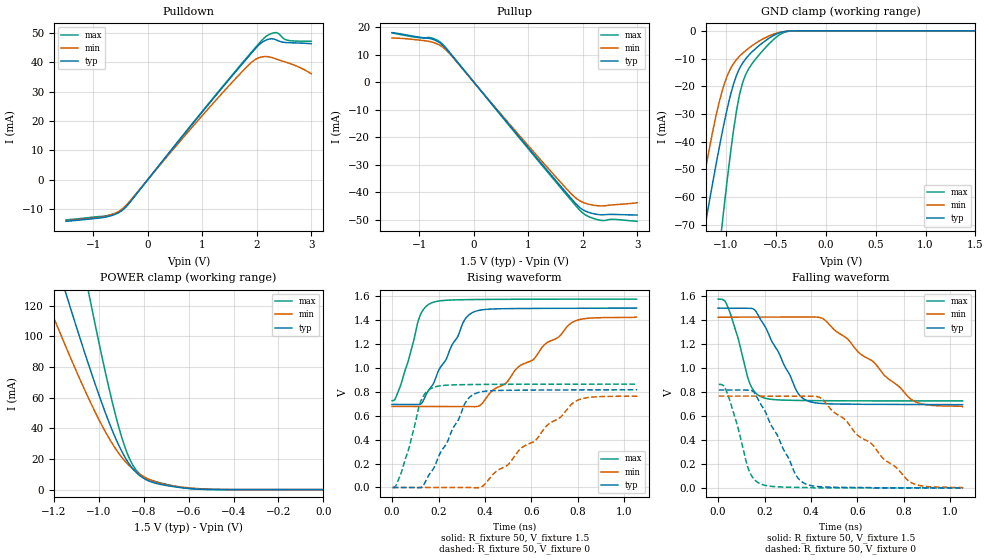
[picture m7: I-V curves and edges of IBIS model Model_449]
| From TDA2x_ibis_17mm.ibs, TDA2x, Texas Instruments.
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| Model based on original model for DDR_DIFFIOPB_H
|   Sub model SR100_DRV40_1P5
[model]   Model_449
|[Description]  [1.5V-I/O-X-X]
|   , ,
|[Input Load]
|[Output Drive]
|Voltage   1.5V
|Mode   I/O
Model_type   I/O
Polarity   Non-Inverting
Enable   Active-Low
Vinl =  0.65
Vinh =  0.85
Cref =  15.0000pF
Rref =  100.0000M
Vref =  0V
Vmeas =  0.75
C_comp   2p   2p   2p
[Model Spec]
Vinl   0.65   0.6125   0.6875
Vinh   0.85   0.8125   0.8875
[Receiver Thresholds]
Tslew_ac = 0.5n
Vth= 0.75
Vth_max= 0.7875
Vth_min= 0.675
Vinh_ac= 0.175
Vinh_dc= 0.1
Vinl_ac= -0.175
Vinl_dc= -0.1
[Temperature Range]   25   125   -40
[Voltage Range]   1.5   1.425   1.575
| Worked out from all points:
|   slope of the pulldown table from 0 to 0.225 V, typ, clamps not added: 43 ohm
|   slope of the pullup table from 0 to 0.225 V, typ, clamps not added: 41.7 ohm
|   GND clamp passes 1 mA (typ) near -0.48 V on its own axis
|   POWER clamp passes 1 mA (typ) near -0.62 V on its own axis
|   rising waveform, R_fixture 50, V_fixture 1.5: 20-80 % time 123ps typ, 282ps min, 71.2ps max; typ from 0.695 V to 1.5 V
|   rising waveform, R_fixture 50, V_fixture 0: 20-80 % time 123ps typ, 273ps min, 71.1ps max; typ from 0 V to 0.817 V
|   falling waveform, R_fixture 50, V_fixture 1.5: 20-80 % time 122ps typ, 255ps min, 70.8ps max; typ from 1.5 V to 0.695 V
|   falling waveform, R_fixture 50, V_fixture 0: 20-80 % time 123ps typ, 263ps min, 71.1ps max; typ from 0.817 V to 0 V
[POWER_clamp]
-1.5V     302.8mA    223.9mA    484.4mA
-1.242V   174.3mA    127.3mA    279.1mA
-1.136V   123.3mA    89.68mA    196.8mA
-1.045V   81.65mA    59.62mA    128.8mA
-1.03V    75mA       54.92mA    117.8mA
-939.4mV  38.44mA    29.91mA    56.84mA
-893.9mV  23.93mA    20.41mA    32.31mA
-848.5mV  13.61mA    13.43mA    15.91mA
-803mV    7.623mA    8.663mA    8.564mA
-712.1mV  3.022mA    3.561mA    3.877mA
-575.8mV  470.5uA    872uA      449uA
0V        112.6nA    435.6nA    613.8nA
[Pulldown]
-1.5V     -14.18mA   -14.05mA   -13.7mA
-727.3mV  -12.54mA   -12.27mA   -12.15mA
-545.5mV  -11.35mA   -10.95mA   -11.1mA
-409.1mV  -9.378mA   -8.925mA   -9.416mA
1.227V    28.16mA    26.58mA    28.43mA
1.818V    41.23mA    38.42mA    41.56mA
2V        45.11mA    41.2mA     45.49mA
2.182V    47.62mA    41.92mA    48.94mA
2.273V    47.99mA    41.65mA    49.78mA
2.364V    47.57mA    41.06mA    50.1mA
2.545V    46.7mA     39.96mA    47.58mA
3V        46.28mA    36.09mA    47.12mA
[Pullup]
-1.5V     17.97mA    16.01mA    17.82mA
-1V       16.28mA    15.23mA    16.1mA
-772.7mV  15.66mA    14.54mA    16.02mA
-590.9mV  13.75mA    12.97mA    14.08mA
-409.1mV  9.799mA    9.534mA    9.955mA
1.409V    -33.42mA   -32.26mA   -33.94mA
1.773V    -41.87mA   -40.19mA   -42.52mA
1.909V    -44.87mA   -42.6mA    -45.68mA
2.091V    -47.15mA   -44.23mA   -48.65mA
2.318V    -48.13mA   -44.93mA   -50.11mA
2.591V    -48.02mA   -44.49mA   -49.82mA
3V        -48.22mA   -43.8mA    -50.51mA
[GND_clamp]
-1.5V     -133.6mA   -115.7mA   -234.3mA
-1.288V   -87.29mA   -67.59mA   -156.8mA
-1.197V   -68.11mA   -48.64mA   -124.4mA
-1.045V   -38.25mA   -22.77mA   -72.51mA
-1.015V   -32.88mA   -19.1mA    -62.74mA
-954.5mV  -23.3mA    -13.72mA   -44.4mA
-863.6mV  -13.6mA    -9.192mA   -23.11mA
-803mV    -10.18mA   -7.193mA   -15.89mA
-681.8mV  -5.771mA   -4.027mA   -9.287mA
-500mV    -1.264mA   -914.7uA   -2.429mA
-348.5mV  -52.39uA   -75.11uA   -85.87uA
1.5V      112.6nA    528.1nA    514.5nA
[Ramp]
dV/dt_f 0.48370113/0.12245937n 0.44921855/0.2558091n 0.51003447/70.870305p
dV/dt_r 0.49166536/0.12309493n 0.46147734/0.27547307n 0.51977443/71.26725p
R_load = 50
[Rising Waveform]
R_fixture = 50
V_fixture = 1.5
V_fixture_min = 1.425
V_fixture_max = 1.575
0s        694.7mV    677.7mV    726.3mV
13.19ps   694.6mV    677.6mV    741.2mV
37.73ps   694mV      677.6mV    859.2mV
119.9ps   695.1mV    677.6mV    1.434V
170.5ps   845.7mV    677.7mV    1.544V
310.2ps   1.394V     677.3mV    1.57V
353.7ps   1.47V      675.6mV    1.572V
489.4ps   1.495V     870.6mV    1.574V
778.3ps   1.499V     1.384V     1.575V
1.053ns   1.5V       1.425V     1.575V
[Rising Waveform]
R_fixture = 50
V_fixture = 0
V_fixture_min = 0
V_fixture_max = 0
2.736ps   0V         0V         0V
40.71ps   0V         0V         130.7mV
123.1ps   0V         0V         718.3mV
173.7ps   144.3mV    0V         833.4mV
315.2ps   708mV      0V         860.2mV
360.9ps   787.7mV    -3.03mV    861.3mV
497.4ps   813mV      187.8mV    863mV
552.2ps   814mV      321.7mV    863.3mV
790.4ps   816mV      721mV      863.9mV
1.055ns   817.1mV    766.1mV    864.1mV
[Falling Waveform]
R_fixture = 50
V_fixture = 1.5
V_fixture_min = 1.425
V_fixture_max = 1.575
0s        1.5V       1.425V     1.575V
36.88ps   1.5V       1.425V     1.532V
83.39ps   1.5V       1.425V     1.267V
133.8ps   1.501V     1.425V     883.8mV
187.3ps   1.39V      1.425V     758.2mV
338.6ps   807.3mV    1.425V     729.9mV
383.6ps   727.2mV    1.426V     728.7mV
458.9ps   702.8mV    1.402V     727.4mV
839.3ps   695.8mV    728.6mV    725.6mV
1.053ns   694.7mV    677.7mV    725.4mV
[Falling Waveform]
R_fixture = 50
V_fixture = 0
V_fixture_min = 0
V_fixture_max = 0
2.736ps   817.1mV    766.1mV    864.1mV
25.57ps   817.2mV    766.1mV    847.5mV
47.12ps   817.2mV    766.1mV    748.9mV
134ps     816.9mV    766.2mV    138.9mV
183.3ps   699.1mV    766.1mV    32.56mV
334.3ps   108.6mV    766mV      3.834mV
377ps     32.82mV    766.4mV    2.645mV
447.4ps   8.582mV    742.6mV    0V
828.5ps   0V         47.07mV    0V
1.055ns   0V         0V         0V
